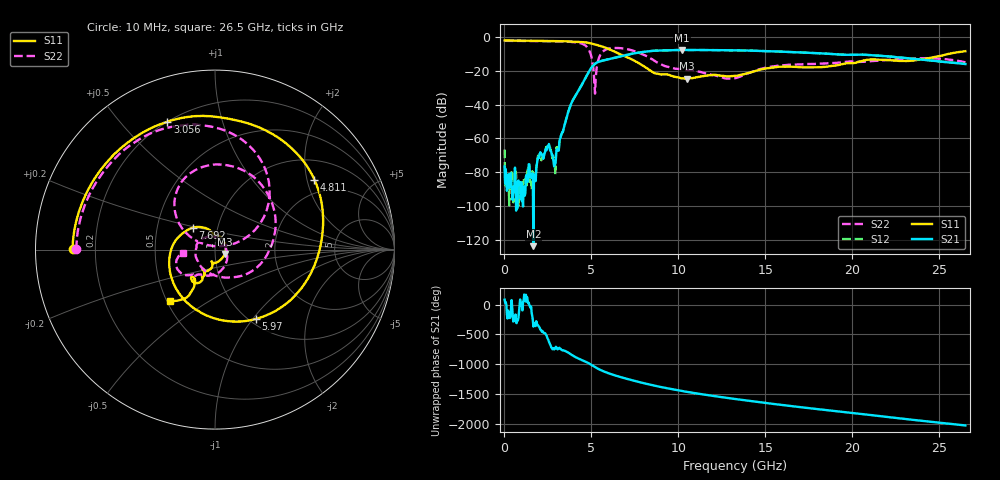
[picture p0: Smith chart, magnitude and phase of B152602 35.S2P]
!  2-Port S-parameters saved by WinCal
! VAR MeasName=S-Parameters (CALIBRATED_DATA) read from VNA (N5242A)
! VAR MeasDate=2016-1-5 16:31:22
! VAR NAME=B152602 35
! VAR FILENAME=B152602 35.S2P
! VAR DATE=2016-1-5 16:31:22
! VAR PHYS_PORTS=1,2
# Hz S DB R 50
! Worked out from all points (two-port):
!   801 points, 10 MHz to 26.5 GHz, reference 50 ohm
!   highest |S21| = -7.62 dB at 10.21 GHz (marker M1); lowest = -123.9 dB at 1.666 GHz (marker M2)
!   |S21| within 3 dB of the highest: 7.001 GHz to 20.89 GHz (13.89 GHz wide, 99.6 % of centre)
!   lowest |S11| = -24.7 dB at 10.51 GHz (marker M3), VSWR 1.12, Z = 55.5 - j2.78 ohm
!   |S11| at or under -10 dB: 6.617 GHz to 25.52 GHz (18.9 GHz wide, 118 % of centre)
!   |S22| runs from -33.5 to -2.2 dB; largest |S21 - S12| = 0.0027
!   S11 on the Smith chart (normalised r, x): 10 MHz: 0.12, +0.00; 3.056 GHz: 0.20, +0.68; 4.811 GHz: 1.55, +2.22; 5.97 GHz: 1.07, -1.04; 7.692 GHz: 0.76, +0.19; 26.5 GHz: 0.52, -0.35
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1e7  -2.01 179.8  -76.64 83.2  -66.61 136.3  -2.24 179.8
1.755625e8  -2.02 176.4  -88.98 128.0  -84.83 -52.4  -2.24 177.3
1.665625e9  -2.19 145.4  -123.92 -6.9  -80.27 -18.8  -2.35 153.9
2.460325e9  -2.29 126.8  -64.71 167.8  -64.50 166.1  -2.44 139.9
2.824562e9  -2.33 117.1  -73.98 -8.4  -72.51 -20.1  -2.48 132.6
3.05635e9  -2.38 110.4  -66.72 -30.0  -65.18 -25.7  -2.53 127.5
3.784825e9  -2.67 85.9  -40.81 -105.1  -40.81 -105.2  -2.84 107.6
4.447075e9  -2.94 56.7  -28.33 153.5  -28.36 153.5  -3.88 78.3
4.811312e9  -3.39 35.1  -21.32 103.7  -21.34 103.8  -6.82 48.2
5.208662e9  -4.39 7.8  -15.83 34.6  -15.83 34.8  -33.55 111.4
5.539788e9  -5.35 -18.2  -14.25 -16.9  -14.24 -16.7  -10.08 135.7
5.97025e9  -6.96 -59.3  -13.13 -67.6  -13.13 -67.6  -6.93 106.7
6.76495e9  -10.67 -144.2  -11.20 -140.7  -11.19 -140.5  -6.66 66.7
7.6921e9  -15.23 135.2  -9.20 147.2  -9.20 147.1  -9.17 16.3
8.851038e9  -21.81 91.6  -7.99 68.9  -7.99 68.9  -15.41 -66.7
1.020865e10  -24.51 -1.4  -7.62 -6.5  -7.63 -6.4  -19.19 -170.2
1.050666e10  -24.66 -25.2  -7.66 -21.5  -7.66 -21.4  -19.66 174.0
1.3255e10  -23.00 -103.3  -7.87 -140.1  -7.87 -140.2  -24.45 9.8
1.577155e10  -17.60 -113.9  -8.57 125.8  -8.58 125.8  -16.90 -95.1
1.769208e10  -17.96 -120.9  -9.41 60.0  -9.38 60.1  -15.97 -119.2
2.209604e10  -13.66 -130.2  -11.52 -84.1  -11.46 -84.4  -13.52 -137.5
2.65e10  -8.37 -131.5  -15.97 136.5  -15.95 136.2  -14.93 -174.3
